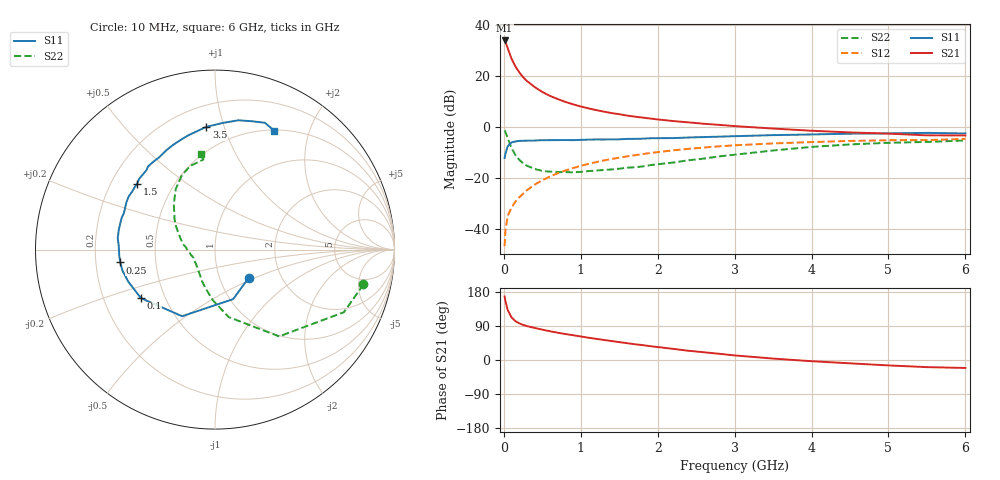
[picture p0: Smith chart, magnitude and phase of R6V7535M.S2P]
! SIEMENS Small Signal Semiconductors
! BFR193
! Si NPN RF Bipolar Junction Transistor in SOT23
! VCE = 0.75 V  IC = 35 mA
! Common Emitter S-Parameters:  May  1996
# GHz  S  MA  R  50
!  f  S11  S21  S12  S22
! GHz  MAG  ANG  MAG  ANG  MAG  ANG  MAG  ANG
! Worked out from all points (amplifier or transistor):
!   36 points, 10 MHz to 6 GHz, reference 50 ohm
!   highest |S21| = 33.8 dB at 10 MHz (marker M1)
!   |S21| within 3 dB of that: start of sweep to 50.04 MHz
!   unconditionally stable (mu >= 1): 311.2 MHz to 2.43 GHz
!   at 250 MHz: K = 0.97, MSG = 22.8 dB, |S12| = -26.2 dB
!   at 1.4 GHz: K = 1.05, MAG = 7.7 dB, |S12| = -12.6 dB
!   at 6 GHz: K = 1.00, MSG = 0.7 dB, |S12| = -4.8 dB
!   S11 on the Smith chart (normalised r, x): 10 MHz: 1.37, -0.46; 100 MHz: 0.37, -0.26; 250 MHz: 0.31, -0.06; 1.5 GHz: 0.31, +0.33; 3.5 GHz: 0.34, +0.87; 6 GHz: 0.51, +1.49
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0.01  0.2448 -39.9  48.92 167.6  0.0046 80.0  0.8498 -13.2
0.02  0.294 -69.9  46.19 156.2  0.0091 74.0  0.7983 -25.9
0.05  0.414 -116.3  34.64 132.0  0.0179 63.5  0.6016 -53.5
0.1  0.4936 -146.8  21.52 112.4  0.0263 61.0  0.3834 -78.6
0.15  0.5154 -159.9  15.2 102.7  0.034 62.9  0.2811 -92.7
0.2  0.5287 -167.2  11.66 96.8  0.0414 65.2  0.226 -102.6
0.25  0.5325 -172.3  9.354 92.7  0.0491 67.1  0.1928 -111.5
0.3  0.5344 -176.1  7.871 89.5  0.0574 68.5  0.1727 -117.7
0.4  0.5373 177.3  5.998 84.6  0.0735 69.5  0.1492 -128.3
0.5  0.5457 173.3  4.797 80.1  0.0899 70.1  0.1369 -137.7
0.6  0.5469 168.8  4.022 75.9  0.1063 69.5  0.132 -144.3
0.7  0.5477 165.0  3.488 72.0  0.1229 68.5  0.1304 -149.6
0.8  0.5492 161.2  3.067 68.6  0.1391 67.3  0.1296 -154.7
0.9  0.5469 158.1  2.749 65.3  0.1556 66.0  0.1283 -159.3
1.1  0.5599 151.7  2.291 58.8  0.1875 63.3  0.1356 -166.2
1.5  0.5676 140.1  1.763 47.2  0.2487 56.9  0.1511 -178.0
2.2  0.6007 121.3  1.294 29.4  0.3453 45.0  0.1992 163.1
3  0.6537 103.2  1.031 12.1  0.4335 31.1  0.2836 142.7
3.5  0.6856 94.1  0.922 3.8  0.4718 23.0  0.3434 131.9
4.5  0.7319 79.8  0.775 -8.8  0.5278 8.9  0.4513 114.3
5.5  0.7595 68.5  0.679 -18.8  0.5487 -4.0  0.5055 97.4
6  0.7397 63.6  0.676 -21.0  0.5786 -7.9  0.5385 98.5
